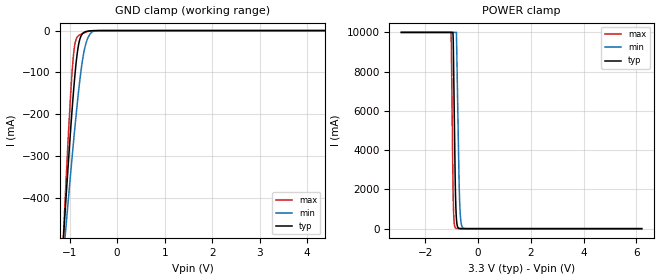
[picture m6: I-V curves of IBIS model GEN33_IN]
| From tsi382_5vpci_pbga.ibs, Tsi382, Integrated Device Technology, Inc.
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|   MODEL GEN33_IN
[Model]   GEN33_IN
Model_type  Input
C_comp 2.4p 2.218p 2.589p
Polarity   Non-Inverting
Enable   Active-High
|   typ   min   max
Vinl   =   0.800v
Vinh   =   2.000v
[Model Spec]
[Temperature Range]   25   125   -40
[Voltage Range] 3.3 3.135 3.465
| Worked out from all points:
|   GND clamp passes 1 mA (typ) near -0.60 V on its own axis
|   POWER clamp passes 1 mA (typ) near -0.61 V on its own axis
[GND Clamp]
-2.907V   -3.934A    -3.096A    -5.193A
-1.157V   -541.7mA   -575.3mA   -550.7mA
-1.104V   -448.3mA   -504.9mA   -425mA
-1.058V   -367.2mA   -443.2mA   -317.4mA
-976.4mV  -232.2mA   -337.9mA   -147.1mA
-912.4mV  -136.9mA   -258.6mA   -51.4mA
-871.7mV  -85.67mA   -210.5mA   -23.35mA
-813.6mV  -34.59mA   -146.6mA   -12.19mA
-697.3mV  -4.311mA   -49.95mA   -5.447mA
-586.8mV  -839.2uA   -11.18mA   -1.549mA
-429.9mV  -53.02uA   -299.5uA   -77.92uA
4.367V    0A         0A         0A
[Power Clamp]
-2.907V   10A        10A        10A
-1.022V   10A        10A        10A
-1.01V    10A        10A        9.399A
-937.4mV  9.599A     10A        1.482A
-901.1mV  6.08A      10A        288.3mA
-852.8mV  1.77A      10A        33.34mA
-816.5mV  488.7mA    10A        10.55mA
-719.9mV  14.04mA    2.643A     3.776mA
-695.7mV  6.492mA    1.421A     3.217mA
-647.4mV  1.907mA    373.7mA    2.245mA
-574.9mV  565.5uA    46.93mA    1.103mA
6.207V    0A         0A         0A
